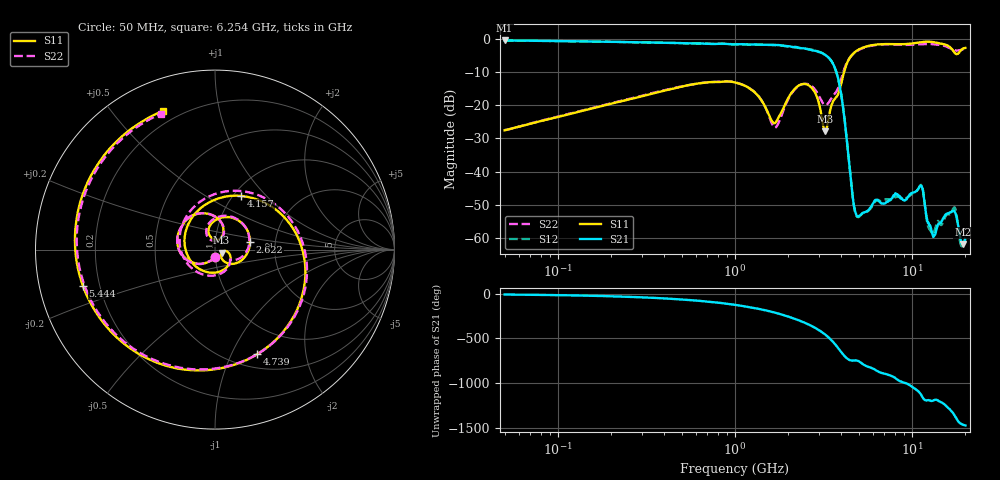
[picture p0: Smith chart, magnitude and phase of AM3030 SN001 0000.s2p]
# Hz S DB R 50
!freq MagS11 AngS11 MagS21 AngS21 MagS12 AngS12 MagS22 AngS22
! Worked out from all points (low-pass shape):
!   1601 points, 50 MHz to 20.05 GHz, reference 50 ohm
!   highest |S21| = -0.41 dB at 50 MHz (marker M1); lowest = -61.9 dB at 19.39 GHz (marker M2)
!   |S21| within 3 dB of the highest: start of sweep to 2.736 GHz
!   lowest |S11| = -27.9 dB at 3.246 GHz (marker M3), VSWR 1.08, Z = 53.8 - j1.81 ohm
!   |S11| at or under -10 dB: start of sweep to 4.134 GHz
!   |S22| runs from -27.4 to -1.5 dB; largest |S21 - S12| = 0.02
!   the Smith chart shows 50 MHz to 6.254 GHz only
!   S11 on the Smith chart (normalised r, x): 50 MHz: 1.00, -0.08; 2.622 GHz: 1.48, +0.13; 4.157 GHz: 1.09, +0.73; 4.739 GHz: 0.65, -1.26; 5.444 GHz: 0.14, -0.13; 6.254 GHz: 0.14, +0.68
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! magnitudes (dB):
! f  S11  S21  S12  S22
! 50 MHz  -27.5  -0.4  -0.4  -27.4
! 135.9 MHz  -21.7  -0.7  -0.7  -21.6
! 369.6 MHz  -16.0  -1.1  -1.1  -15.8
! 1.005 GHz  -13.1  -1.6  -1.6  -13.1
! 1.336 GHz  -16.8  -1.6  -1.7  -16.8
! 1.685 GHz  -25.3  -1.8  -1.8  -26.7
! 2.142 GHz  -15.5  -2.4  -2.5  -15.6
! 2.622 GHz  -14.0  -3.1  -3.1  -13.7
! 2.722 GHz  -14.8  -3.4  -3.2  -14.3
! 3.246 GHz  -27.9  -4.8  -4.8  -19.9
! 3.757 GHz  -17.4  -10.2  -10.3  -15.7
! 4.157 GHz  -9.6  -23.9  -23.7  -8.9
! 4.739 GHz  -4.0  -51.2  -51.4  -4.1
! 5.444 GHz  -2.3  -52.2  -52.3  -2.5
! 6.254 GHz  -1.7  -48.5  -48.8  -1.8
! 7.402 GHz  -1.5  -48.7  -48.5  -1.6
! 11.22 GHz  -0.9  -44.2  -44.0  -1.5
! 12.79 GHz  -0.8  -56.9  -57.8  -1.5
! 13.38 GHz  -1.0  -59.3  -58.1  -1.6
! 17.32 GHz  -3.9  -51.9  -50.8  -3.3
! 19.39 GHz  -2.9  -61.9  -62.1  -3.1
! 20.05 GHz  -2.7  -60.4  -60.0  -3.1
